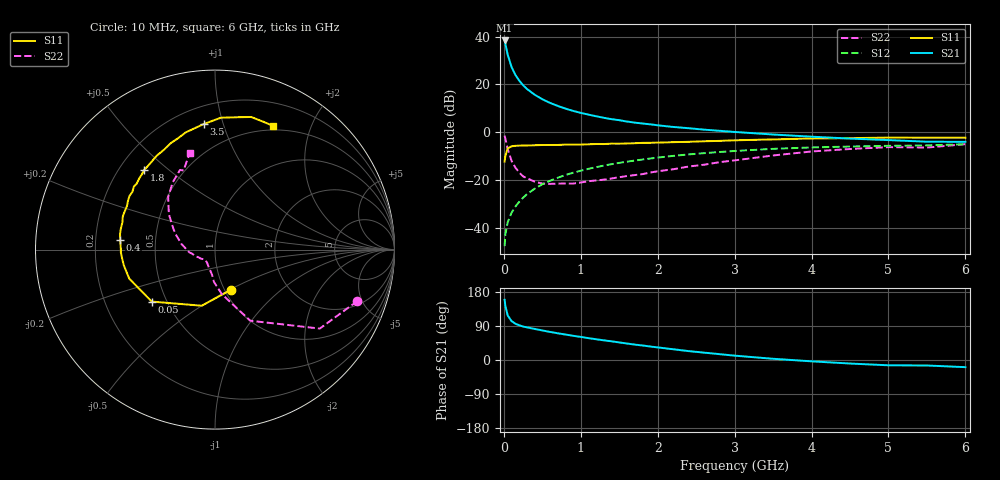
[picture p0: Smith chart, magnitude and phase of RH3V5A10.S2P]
! SIEMENS Small Signal Semiconductors
! BFR106
! Si NPN RF Bipolar Junction Transistor in SOT23
! VCE = 3.5 V  IC = 100 mA
! Common Emitter S-Parameters:  August  1996
# GHz  S  MA  R  50
!  f  S11  S21  S12  S22
! GHz  MAG  ANG  MAG  ANG  MAG  ANG  MAG  ANG
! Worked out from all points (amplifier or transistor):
!   36 points, 10 MHz to 6 GHz, reference 50 ohm
!   highest |S21| = 38.3 dB at 10 MHz (marker M1)
!   |S21| within 3 dB of that: start of sweep to 30.47 MHz
!   unconditionally stable (mu >= 1): 151.1 MHz to 2.65 GHz; 5.281 GHz to end of sweep
!   at 250 MHz: K = 1.08, MAG = 21.8 dB, |S12| = -27.5 dB
!   at 1.4 GHz: K = 1.07, MAG = 7.8 dB, |S12| = -13.4 dB
!   at 6 GHz: K = 1.01, MAG = 0.0 dB, |S12| = -5.1 dB
!   S11 on the Smith chart (normalised r, x): 10 MHz: 1.07, -0.51; 50 MHz: 0.41, -0.30; 400 MHz: 0.31, +0.04; 1.8 GHz: 0.30, +0.42; 3.5 GHz: 0.31, +0.86; 6 GHz: 0.45, +1.47
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0.01  0.2411 -68.3  82.65 158.8  0.0041 76.9  0.8433 -19.9
0.02  0.3214 -103.3  70.21 142.8  0.0073 70.4  0.7311 -37.0
0.05  0.4562 -140.6  41.66 117.5  0.013 59.7  0.4424 -63.6
0.1  0.5044 -161.3  23.09 102.7  0.0205 65.6  0.251 -81.3
0.15  0.5157 -170.3  15.72 95.8  0.0276 69.1  0.1805 -91.8
0.2  0.5197 -174.4  11.96 91.7  0.0347 71.8  0.1428 -96.4
0.25  0.5247 -178.3  9.559 88.4  0.0424 72.5  0.1186 -103.2
0.3  0.5249 179.1  8.007 86.1  0.0501 73.9  0.1085 -107.8
0.4  0.5305 174.4  6.063 82.0  0.0652 74.2  0.0919 -116.1
0.5  0.5364 170.5  4.868 78.0  0.0807 73.7  0.0837 -122.4
0.6  0.5375 167.3  4.084 74.1  0.0958 72.6  0.0823 -126.9
0.7  0.538 163.4  3.529 70.5  0.1107 71.7  0.0837 -132.0
0.9  0.5462 157.3  2.776 63.9  0.1411 69.1  0.0836 -141.0
1.1  0.5558 150.7  2.321 57.7  0.1704 66.0  0.0938 -147.5
1.4  0.5723 142.2  1.866 49.3  0.2128 61.5  0.107 -157.6
1.8  0.5947 131.5  1.515 38.4  0.2664 55.1  0.1317 -170.6
2.2  0.6156 121.9  1.281 28.4  0.3173 48.6  0.1665 176.9
2.8  0.6536 108.3  1.065 15.5  0.3828 38.8  0.2342 159.0
3.5  0.7021 95.2  0.89 3.2  0.4462 27.9  0.3241 142.5
4.5  0.7475 80.6  0.731 -9.3  0.4986 13.3  0.4427 122.1
5.5  0.7614 69.0  0.629 -14.5  0.5265 4.1  0.4745 111.7
6  0.7613 65.0  0.625 -18.9  0.5582 -2.8  0.5583 104.5
